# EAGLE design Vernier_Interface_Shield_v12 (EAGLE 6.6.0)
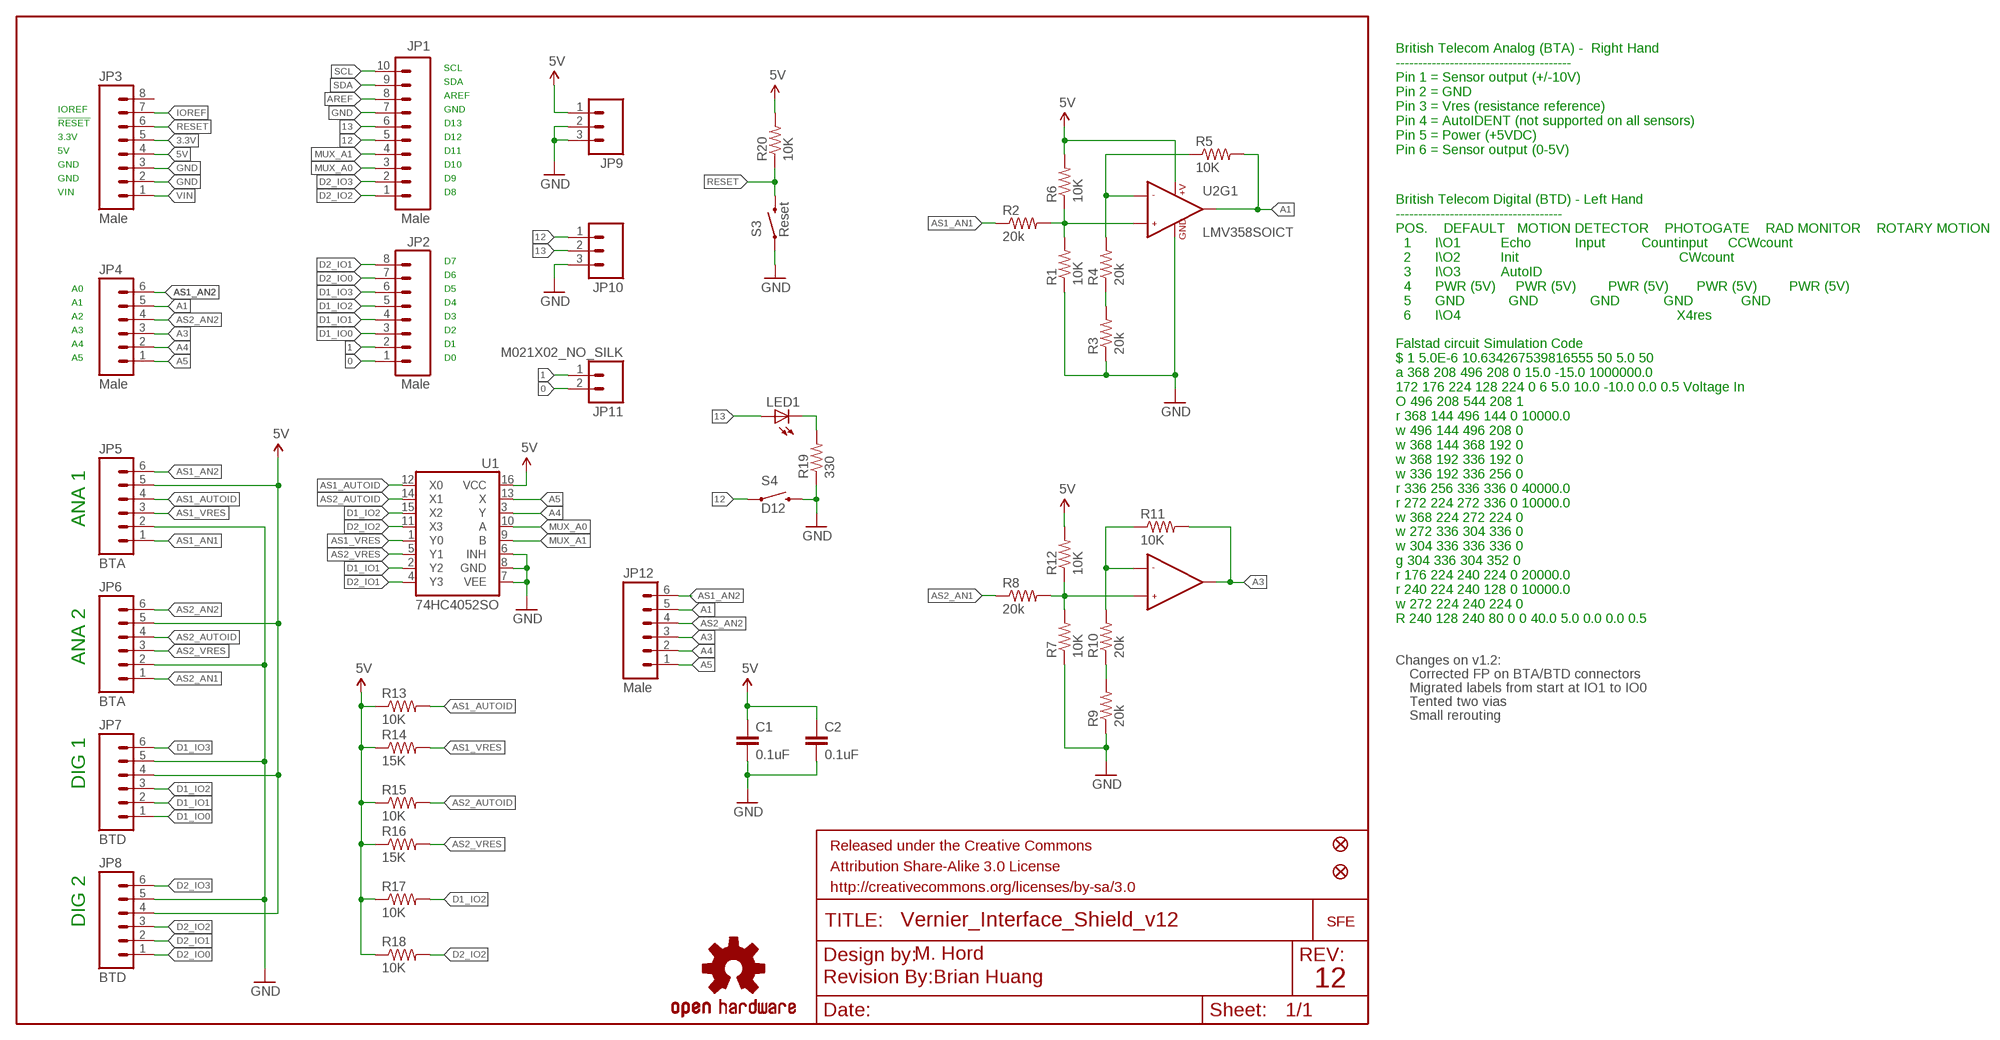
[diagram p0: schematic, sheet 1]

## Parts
C1  0.1uF  0.1UF-25V(+80/-20%)(0603)  [0603-CAP]
C2  0.1uF  0.1UF-25V(+80/-20%)(0603)  [0603-CAP]
FID1  FIDUCIAL1X2  [FIDUCIAL-1X2]
FID2  FIDUCIAL1X2  [FIDUCIAL-1X2]
FRAME1  FRAME-LETTER  [CREATIVE_COMMONS]
JP1  Male  M10SMD_MALE  [1X10_SMD_MALE]
JP2  Male  M08SMD-MALE  [1X08_SMD_MALE]
JP3  Male  M08SMD-MALE  [1X08_SMD_MALE]
JP4  Male  M06SMD_MALE  [1X06_SMD_MALE]
JP5  BTA  M06VERNIER-ANALOG  [BTA]
JP6  BTA  M06VERNIER-ANALOG  [BTA]
JP7  BTD  M06VERNIER-DIGITAL  [BTD]
JP8  BTD  M06VERNIER-DIGITAL  [BTD]
JP9  M031X03_NO_SILK  [1X03_NO_SILK]
JP10  M031X03_NO_SILK  [1X03_NO_SILK]
JP11  M021X02_NO_SILK  [1X02_NO_SILK]
JP12  Male  M06SIP  [1X06]
LED1  LED5MM  [LED5MM]
LOGO2  OSHW-LOGOS  [OSHW-LOGO-S]
LOGO_1  LOGO-SFESK  [SFE-LOGO-FLAME]
R1  10K  10KOHM1/10W1%(0603)0603  [0603-RES]
R2  20k  20KOHM1/10W1%(0603)  [0603-RES]
R3  20k  20KOHM1/10W1%(0603)  [0603-RES]
R4  20k  20KOHM1/10W1%(0603)  [0603-RES]
R5  10K  10KOHM1/10W1%(0603)0603  [0603-RES]
R6  10K  10KOHM1/10W1%(0603)0603  [0603-RES]
R7  10K  10KOHM1/10W1%(0603)0603  [0603-RES]
R8  20k  20KOHM1/10W1%(0603)  [0603-RES]
R9  20k  20KOHM1/10W1%(0603)  [0603-RES]
R10  20k  20KOHM1/10W1%(0603)  [0603-RES]
R11  10K  10KOHM1/10W1%(0603)0603  [0603-RES]
R12  10K  10KOHM1/10W1%(0603)0603  [0603-RES]
R13  10K  10KOHM1/10W1%(0603)0603  [0603-RES]
R14  15K  15KOHM1/10W1%(0603)0603  [0603-RES]
R15  10K  10KOHM1/10W1%(0603)0603  [0603-RES]
R16  15K  15KOHM1/10W1%(0603)0603  [0603-RES]
R17  10K  10KOHM1/10W1%(0603)0603  [0603-RES]
R18  10K  10KOHM1/10W1%(0603)0603  [0603-RES]
R19  330  330OHM1/10W1%(0603)  [0603-RES]
R20  10K  10KOHM1/10W1%(0603)0603  [0603-RES]
S3  Reset  SWITCH-MOMENTARY-2PTH  [TACTILE-PTH]
S4  D12  SWITCH-MOMENTARY-2PTH  [TACTILE-PTH]
U1  74HC4052SO  [SO16]
U2  LMV358SOICT  [SO08-TIGHT]
U$1  REVISION  [REVISION]

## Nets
0: JP2.1 JP11.2
1: JP2.2 JP11.1
3.3V: JP3.5
5V: C1.1 C2.1 JP3.4 JP5.5 JP6.5 JP7.4 JP8.4 JP9.1 R6.2 R12.2 R13.1 R14.1 R15.1 R16.1 R17.1 R18.1 R20.2 U1.16(VCC) U2.8(+V)
12: JP1.5 JP10.1 S4.1
13: JP1.6 JP10.2 LED1.A
A1: JP4.5 JP12.5 R5.2 U2.1(OUT1)
A3: JP4.3 JP12.3 R11.2 U2.7(OUT2)
A4: JP4.2 JP12.2 U1.3(Y)
A5: JP4.1 JP12.1 U1.13(X)
AREF: JP1.8
AS1_AN1: JP5.1 R2.1
AS1_AN2: JP4.6 JP5.6 JP12.6
AS1_AUTOID: JP5.4 R13.2 U1.12(X0)
AS1_VRES: JP5.3 R14.2 U1.1(Y0)
AS2_AN1: JP6.1 R8.1
AS2_AN2: JP4.4 JP6.6 JP12.4
AS2_AUTOID: JP6.4 R15.2 U1.14(X1)
AS2_VRES: JP6.3 R16.2 U1.5(Y1)
D1_IO0: JP2.3 JP7.1
D1_IO1: JP2.4 JP7.2 U1.2(Y2)
D1_IO2: JP2.5 JP7.3 R17.2 U1.15(X2)
D1_IO3: JP2.6 JP7.6
D2_IO0: JP2.7 JP8.1
D2_IO1: JP2.8 JP8.2 U1.4(Y3)
D2_IO2: JP1.1 JP8.3 R18.2 U1.11(X3)
D2_IO3: JP1.2 JP8.6
GND: C1.2 C2.2 JP1.7 JP3.2 JP3.3 JP5.2 JP6.2 JP7.5 JP8.5 JP9.2 JP9.3 JP10.3 R1.1 R3.1 R7.1 R9.1 R19.1 S3.1 S4.3 U1.6(INH) U1.7(VEE) U1.8(GND) U2.4(GND)
IOREF: JP3.7
MUX_A0: JP1.3 U1.10(A)
MUX_A1: JP1.4 U1.9(B)
N$1: R1.2 R2.2 R6.1 U2.3(+IN1)
N$2: R3.2 R4.1
N$3: R4.2 R5.1 U2.2(-IN1)
N$5: R9.2 R10.1
N$6: R7.2 R8.2 R12.1 U2.5(+IN2)
N$8: R10.2 R11.1 U2.6(-IN2)
N$9: LED1.K(C) R19.2
RESET: JP3.6 R20.1 S3.3
SCL: JP1.10
SDA: JP1.9
VIN: JP3.1
Unconnected: JP3.8

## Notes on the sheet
- SCL
- SDA
- AREF
- IOREF | GND
- !RESET | D13
- 3.3V | D12
- 5V | D11
- British Telecom Analog (BTA) -  Right Hand
  ---------------------------------------
  Pin 1 = Sensor output (+/-10V)
  Pin 2 = GND
  Pin 3 = Vres (resistance reference)
  Pin 4 = AutoIDENT (not supported on all sensors)
  Pin 5 = Power (+5VDC)
  Pin 6 = Sensor output (0-5V)
- GND | D10
- GND | D9
- VIN | D8
- D7
- D6
- A0 | D5
- A1 | D4
- A2 | D3
- British Telecom Digital (BTD) - Left Hand
  -------------------------------------
  POS.    DEFAULT   MOTION DETECTOR    PHOTOGATE    RAD MONITOR    ROTARY MOTION
    1      I\\O1          Echo           Input         Countinput     CCWcount 
    2      I\\O2          Init                                        CWcount 
    3      I\\O3          AutoID            
    4      PWR (5V)     PWR (5V)        PWR (5V)       PWR (5V)        PWR (5V)
    5      GND           GND             GND           GND            GND
    6      I\\O4                                                      X4res
- A3 | D2
- A4 | D1
- A5 | D0
- ANA 1
- Falstad circuit Simulation Code
  $ 1 5.0E-6 10.634267539816555 50 5.0 50
  a 368 208 496 208 0 15.0 -15.0 1000000.0
  172 176 224 128 224 0 6 5.0 10.0 -10.0 0.0 0.5 Voltage In
  O 496 208 544 208 1
  r 368 144 496 144 0 10000.0
  w 496 144 496 208 0
  w 368 144 368 192 0
  w 368 192 336 192 0
  w 336 192 336 256 0
  r 336 256 336 336 0 40000.0
  r 272 224 272 336 0 10000.0
  w 368 224 272 224 0
  w 272 336 304 336 0
  w 304 336 336 336 0
  g 304 336 304 352 0
  r 176 224 240 224 0 20000.0
  r 240 224 240 128 0 10000.0
  w 272 224 240 224 0
  R 240 128 240 80 0 0 40.0 5.0 0.0 0.0 0.5
- ANA 2 | Changes on v1.2:
- Corrected FP on BTA/BTD connectors
- Migrated labels from start at IO1 to IO0
- Tented two vias
- Small rerouting
- DIG 1
- DIG 2
- M. Hord
- Brian Huang | 12

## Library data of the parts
C1 C2 = SparkFun-Capacitors:0.1UF-25V(+80/-20%)(0603): CAP-00810; PROD_ID: CAP-00810
FID1 FID2 = SparkFun-Aesthetics:FIDUCIAL: Fiducial Alignment Points
FRAME1 = SparkFun-Aesthetics:FRAME-LETTER: Schematic Frame
JP1 = SparkFun-Connectors:M10: Header 10 Standard 10-pin 0.1" header. Use with straight break away headers (SKU : PRT-00116), right angle break away headers (PRT-00553), swiss pins (PRT-00743), machine pins (PRT-00117), and female headers (PRT-00115).; PROD_ID: CONN-11291
JP2 JP3 = SparkFun-Connectors:M08: Header 8 Standard 8-pin 0.1" header. Use with straight break away headers (SKU : PRT-00116), right angle break away headers (PRT-00553), swiss pins (PRT-00743), machine pins (PRT-00117), and female headers (PRT-00115).; PROD_ID: CONN-11292
JP4 = SparkFun-Connectors:M06: Header 6 Standard 6-pin 0.1" header. Use with straight break away headers (SKU : PRT-00116), right angle break away headers (PRT-00553), swiss pins (PRT-00743), machine pins (PRT-00117), and female headers (PRT-00115). Molex polarized connector foot print use with SKU : PRT-08094 with associated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; PROD_ID: CONN-11293
JP5-JP8 JP12 = SparkFun-Connectors:M06: Header 6 Standard 6-pin 0.1" header. Use with straight break away headers (SKU : PRT-00116), right angle break away headers (PRT-00553), swiss pins (PRT-00743), machine pins (PRT-00117), and female headers (PRT-00115). Molex polarized connector foot print use with SKU : PRT-08094 with associated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
JP9 JP10 = SparkFun-Connectors:M03: Header 3 Standard 3-pin 0.1" header. Use with straight break away headers (SKU : PRT-00116), right angle break away headers (PRT-00553), swiss pins (PRT-00743), machine pins (PRT-00117), and female headers (PRT-00115). Molex polarized connector foot print use with SKU : PRT-08232 with associated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
JP11 = SparkFun-Connectors:M02: Standard 2-pin 0.1" header. Use with
LED1 = SparkFun-LED:LED: LEDs
LOGO2 = SparkFun-Aesthetics:OSHW-LOGO: Open Source Hardware Logo This logo indicates the piece of hardware it is found on incorporates a OSHW license and/or adheres to the definition of open source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
LOGO_1 = SparkFun-Aesthetics:LOGO-SFE: Spark Fun Electronics PCB Logo
R1 R5-R7 R11-R13 R15 R17 R18 R20 = SparkFun-Resistors:10KOHM1/10W1%(0603): RES-00824; PROD_ID: RES-00824
R2-R4 R8-R10 = SparkFun-Resistors:20KOHM1/10W1%(0603): RES-09383; PROD_ID: RES-09383
R14 R16 = SparkFun-Resistors:15KOHM1/10W1%(0603): RES-07854; PROD_ID: RES-07854
R19 = SparkFun-Resistors:330OHM1/10W1%(0603): RES-00818; PROD_ID: RES-00818
S3 S4 = SparkFun-Electromechanical:SWITCH-MOMENTARY-2: Various NO switches- pushbuttons, reed, etc
U1 = SparkFun-AnalogIC:74HC4052: Dual 4:1 analog mux; PROD_ID: IC-09813; VALUE: 74HC4052
U2 = SparkFun-AnalogIC:LMV358: Jellybean rail-to-rail output op-amp; PROD_ID: IC-09657
U$1 = SparkFun-Aesthetics:REVISION

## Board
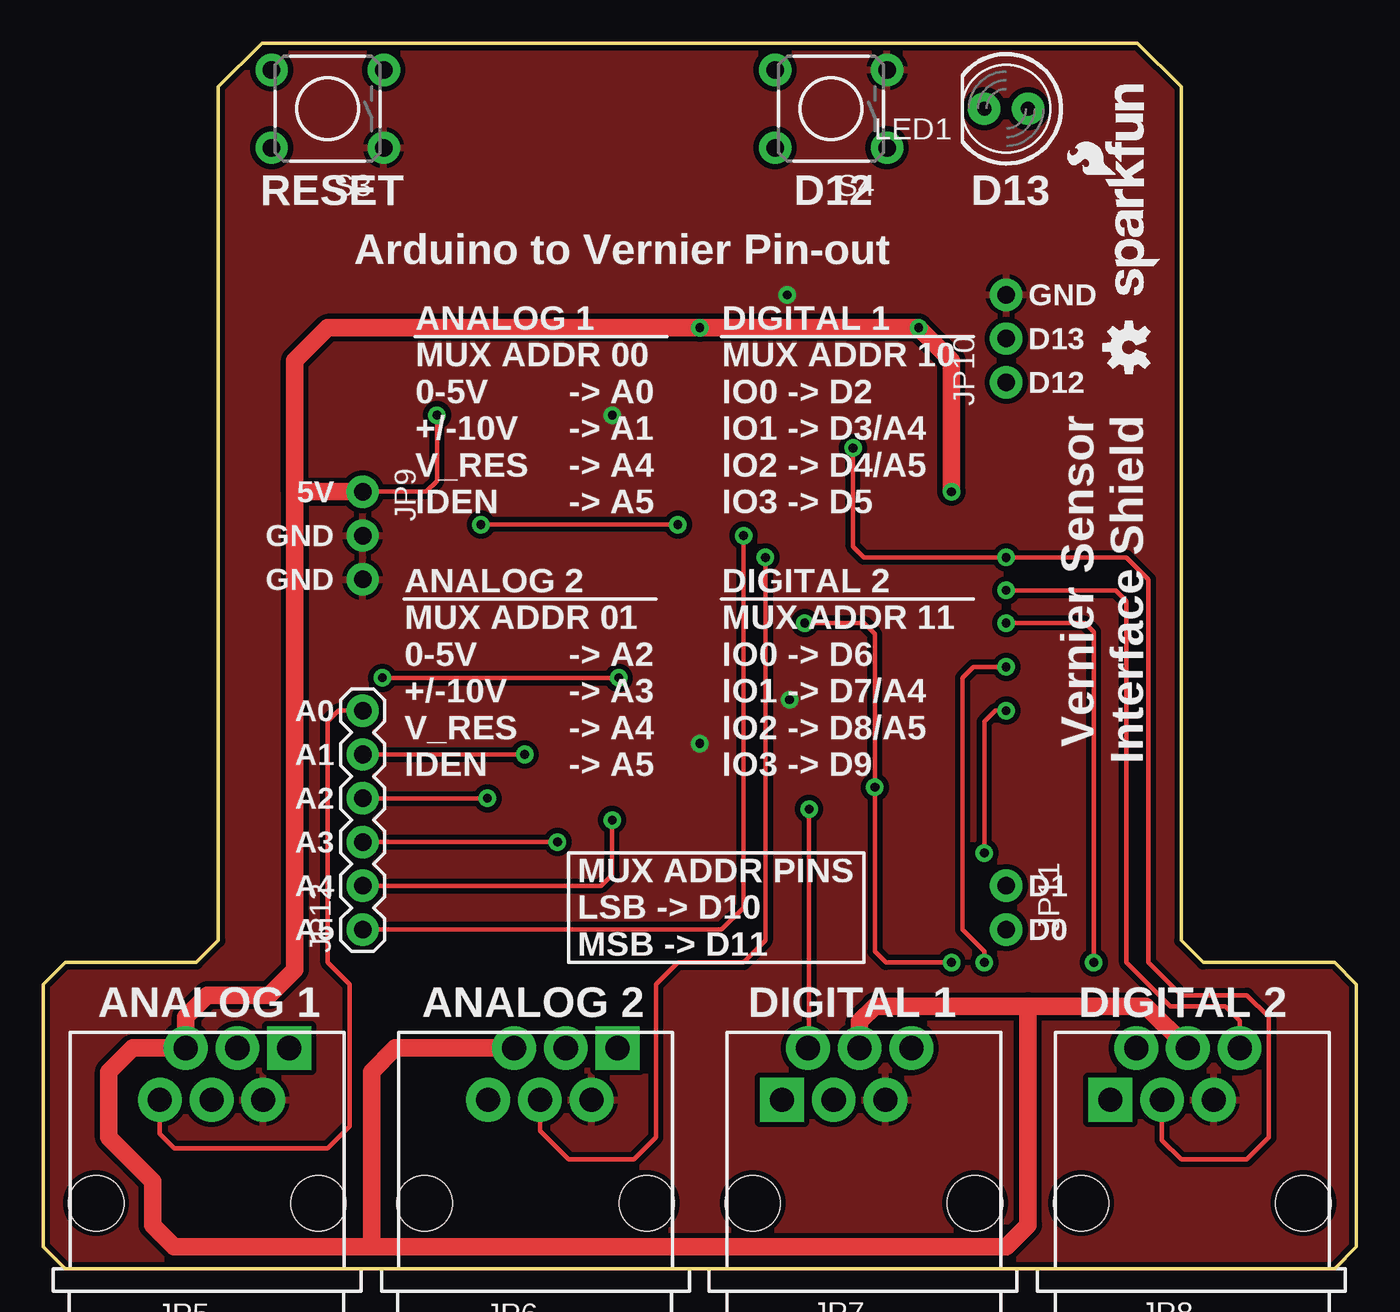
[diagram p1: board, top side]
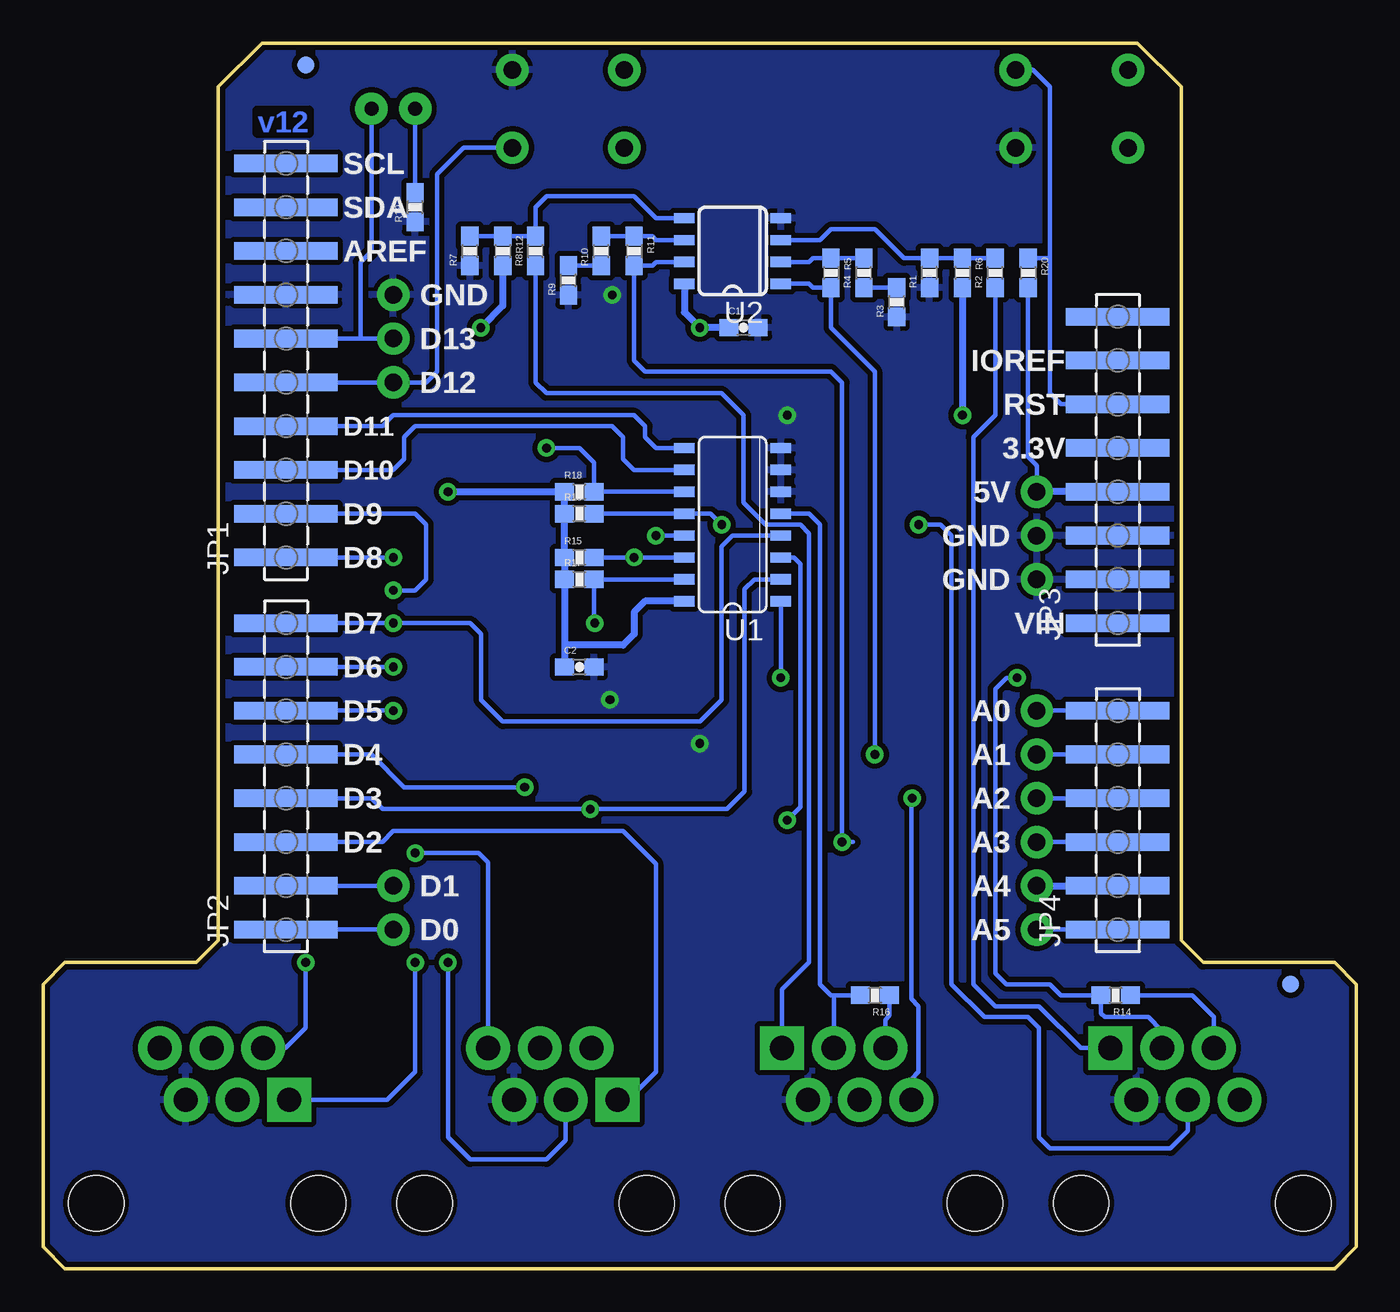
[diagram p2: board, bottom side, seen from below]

Size 76.2 x 71.12 mm. Coordinates in mm from the lower left corner, seen from the top.
Outline: 1.27,0 74.93,0 76.2,1.27 76.2,16.51 74.93,17.78 67.31,17.78 66.04,19.05 66.04,68.58 63.5,71.12 12.7,71.12 10.16,68.58 10.16,19.05 8.89,17.78 1.27,17.78 0,16.51 0,1.27 1.27,0
Copper layers (1*16): Top 0.035mm / dielectric 1.5mm / Bottom 0.035mm
Design rules "SparkFun-2-layer": minimum track width 7mil, minimum drill 15mil, track to track 8mil, track to pad 8mil, pad to pad 8mil, via to via 8mil, smd to smd 8mil, copper to edge 8mil, drill to drill 8mil, minimum pad ring 12mil, minimum via ring 10mil, stop-mask expansion 4mil, vias tented up to drill 20mil, thermal gap 10mil

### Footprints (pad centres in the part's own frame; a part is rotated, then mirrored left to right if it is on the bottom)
0603-CAP = smd 1.1 x 1: 1 -0.85,0; 2 0.85,0
FIDUCIAL-1X2 = smd 1 x 1: 1 0,0
1X10_SMD_MALE = smd 1.02 x 6: 1 0,0; 2 2.54,0; 3 5.08,0; 4 7.62,0; 5 10.16,0; 6 12.7,0; 7 15.24,0; 8 17.78,0; 9 20.32,0; 10 22.86,0
1X08_SMD_MALE = smd 1.02 x 6: 1 0,0; 2 2.54,0; 3 5.08,0; 4 7.62,0; 5 10.16,0; 6 12.7,0; 7 15.24,0; 8 17.78,0
1X06_SMD_MALE = smd 1.02 x 6: 1 0,0; 2 2.54,0; 3 5.08,0; 4 7.62,0; 5 10.16,0; 6 12.7,0
BTA = drill 1.4 pad 2.54 square: 1 4.75,9 | drill 1.4 pad 2.54: 2 3.25,6; 3 1.75,9; 4 0.25,6; 5 -1.25,9; 6 -2.75,6 | hole 3.2: 6.45,0; -6.45,0
BTD = drill 1.4 pad 2.54 square: 1 -4.75,6 | drill 1.4 pad 2.54: 2 -3.25,9; 3 -1.75,6; 4 -0.25,9; 5 1.25,6; 6 2.75,9 | hole 3.2: 6.45,0; -6.45,0
1X03_NO_SILK = drill 1.016 pad 1.88: 1 0,0; 2 2.54,0; 3 5.08,0
1X02_NO_SILK = drill 1.016 pad 1.88: 1 0,0; 2 2.54,0
1X06 = drill 1.016 pad 1.88: 1 0,0; 2 2.54,0; 3 5.08,0; 4 7.62,0; 5 10.16,0; 6 12.7,0
LED5MM = drill 0.813 pad 1.88: A -1.27,0; K 1.27,0
0603-RES = smd 1.1 x 1: 1 -0.85,0; 2 0.85,0
TACTILE-PTH = drill 1.016 pad 1.88: 1 -3.251,2.261; 2 3.251,2.261; 3 -3.251,-2.261; 4 3.251,-2.261
SO16 = smd 0.6 x 1.2: 1 -4.445,-2.8; 2 -3.175,-2.8; 3 -1.905,-2.8; 4 -0.635,-2.8; 5 0.635,-2.8; 6 1.905,-2.8; 7 3.175,-2.8; 8 4.445,-2.8; 9 4.445,2.8; 10 3.175,2.8; 11 1.905,2.8; 12 0.635,2.8; 13 -0.635,2.8; 14 -1.905,2.8; 15 -3.175,2.8; 16 -4.445,2.8
SO08-TIGHT = smd 0.6 x 1.2: 1 -1.905,-2.8; 2 -0.635,-2.8; 3 0.635,-2.8; 4 1.905,-2.8; 5 1.905,2.8; 6 0.635,2.8; 7 -0.635,2.8; 8 -1.905,2.8

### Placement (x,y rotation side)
C1  35.56,54.61 0 bottom
C2  45.09,34.92 0 bottom
FID1  3.81,16.51 0 bottom
FID2  60.96,69.85 0 bottom
FRAME1  not placed on the board
JP1  62.1,41.27 90 bottom
JP2  62.1,19.68 90 bottom
JP3  13.84,37.47 90 bottom
JP4  13.84,19.68 90 bottom
JP5  9.53,3.81 0 top
JP6  28.57,3.81 0 top
JP7  47.62,3.81 0 top
JP8  66.67,3.81 0 top
JP9  18.54,45.09 270 top
JP10  55.88,51.44 90 top
JP11  55.88,22.23 270 top
JP12  18.54,19.68 90 top
LED1  55.88,67.31 180 top
LOGO2  62.99,53.47 90 top
LOGO_1  62.23,63.5 90 top
LOGO_3  LOGO-SFENW2  [SFE-NEW-WEB]  64.77,56.52 90 top
R1  24.77,57.78 90 bottom
R2  20.95,57.78 90 bottom
R3  26.67,56.08 90 bottom
R4  28.57,57.78 90 bottom
R5  30.48,57.78 270 bottom
R6  22.86,57.78 270 bottom
R7  51.44,59.05 90 bottom
R8  47.62,59.05 90 bottom
R9  45.72,57.35 90 bottom
R10  43.81,59.05 90 bottom
R11  41.91,59.05 270 bottom
R12  49.53,59.05 270 bottom
R13  45.09,43.81 0 bottom
R14  13.97,15.88 180 bottom
R15  45.09,41.27 0 bottom
R16  27.94,15.88 180 bottom
R17  45.09,40.01 0 bottom
R18  45.09,45.09 0 bottom
R19  54.61,61.59 90 bottom
R20  19.05,57.78 270 bottom
S3  16.51,67.31 180 top
S4  45.72,67.31 180 top
U1  36.2,43.18 90 bottom
U2  36.2,59.05 90 bottom
U$1  not placed on the board

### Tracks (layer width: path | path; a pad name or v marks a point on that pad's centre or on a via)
0
  Bottom 0.254: JP2.1 JP11.2
1
  Bottom 0.254: JP2.2 JP11.1
5V  (via drill 0.51)
  Top 0.254: JP9.1 22.23,45.09 22.86,45.72 v22.86,49.53
  Top 1.016: 14.61,45.09 JP9.1 | 57.15,15.24 48.26,15.24 47.38,14.36 JP7.4 | 57.15,15.24 63.99,15.24 JP8.4 | JP6.5 20.43,12.81 19.05,11.43 19.05,1.27 | 19.05,1.27 7.62,1.27 6.35,2.54 6.35,5.08 3.81,7.62 3.81,11.43 5.19,12.81 JP5.5 8.28,14.62 9.53,15.88 R14.1 14.61,17.36 14.61,45.09 | 19.05,1.27 55.88,1.27 57.15,2.54 57.15,15.24 | 14.61,45.09 14.61,52.7 16.51,54.61 v38.1,54.61 v50.8,54.61 52.7,52.7 v52.7,45.09
  Bottom 0.254: R14.1 9.53,15.88 8.28,14.62 JP5.5 | JP6.5 27.32,14.46 27.09,14.69 R16.1 | R20.2 19.05,47.12 18.54,46.61 JP9.1
  Bottom 0.406: 45.94,36.2 R17.1 R15.1 R13.1 R18.1 v52.7,45.09 | 45.94,36.2 C2.1 | U1.16 41.27,38.73 41.91,38.1 41.91,36.83 42.55,36.2 45.94,36.2 | R6.2 v22.86,49.53 | C1.1 v38.1,54.61 38.99,55.51 U2.8 | JP3.4 JP9.1 | R12.2 49.53,55.88 v50.8,54.61
12
  Bottom 0.254: JP1.5 JP10.1 53.98,51.44 53.34,52.07 53.34,63.5 51.79,65.05 S4.1
13
  Bottom 0.254: JP1.6 57.78,53.98 | 57.78,53.98 JP10.2 | LED1.A 57.15,59.05 57.78,58.42 57.78,53.98
A1  (via drill 0.51)
  Top 0.254: JP12.5 v27.94,29.84
  Bottom 0.254: v27.94,29.84 27.94,52.07 30.48,54.61 R5.2 31.54,56.94 31.75,57.15 U2.1 | JP4.5 JP12.5
A3  (via drill 0.51)
  Top 0.254: JP12.3 v29.84,24.77
  Bottom 0.254: U2.7 40.64,58.42 40.85,58.2 R11.2 41.91,52.7 41.27,52.07 30.48,52.07 29.84,51.44 v29.84,24.77 29.21,24.77 | JP4.3 JP12.3
A4  (via drill 0.51)
  Top 0.254: JP12.2 32.38,22.23 33.02,22.86 v33.02,26.04
  Bottom 0.254: U1.3 32.64,41.27 32.26,40.89 32.26,26.8 v33.02,26.04
  Bottom 0.406: JP12.2 JP4.2
A5  (via drill 0.51)
  Top 0.254: v40.64,42.55 40.64,20.95 39.37,19.68 JP12.1
  Bottom 0.254: U1.13 v40.64,42.55 | JP12.1 JP4.1
AS1_AN1
  Bottom 0.254: R2.1 20.95,49.53 22.23,48.26 22.23,16.51 20.95,15.24 18.41,15.24 15.98,12.81 JP5.1
AS1_AN2
  Top 0.254: JP5.6 6.78,7.83 7.62,6.99 16.51,6.99 17.78,8.26 17.78,16.51 16.51,17.78 16.51,31.75 17.14,32.38 JP12.6
  Bottom 0.254: JP12.6 JP4.6
AS1_AUTOID  (via drill 0.51)
  Top 0.254: v36.83,43.18 v25.4,43.18
  Bottom 0.254: R13.2 U1.12 37.47,43.81 v36.83,43.18 | JP5.4 9.78,8.01 10.79,6.99 17.78,6.99 18.41,7.62 18.41,13.97 19.05,14.61 21.59,14.61 23.5,16.51 23.5,42.55 24.13,43.18 v25.4,43.18
AS1_VRES  (via drill 0.51)
  Top 0.254: v19.68,34.29 v33.4,34.29
  Bottom 0.254: JP5.3 11.28,13.81 12.06,14.61 14.61,14.61 14.82,14.82 R14.2 17.14,15.88 17.78,16.51 20.32,16.51 20.95,17.14 20.95,33.66 20.32,34.29 v19.68,34.29 | U1.1 v33.4,34.3 v33.4,34.29
AS2_AN1
  Bottom 0.254: R8.1 47.62,51.44 46.99,50.8 36.83,50.8 35.56,49.53 35.56,44.45 34.29,43.18 32.26,43.18 31.75,42.67 31.75,17.78 33.33,16.2 JP6.1
AS2_AN2  (via drill 0.51)
  Top 0.254: JP12.4 v25.78,27.3
  Bottom 0.254: JP4.4 JP12.4 | v25.78,27.3 25.82,27.26 25.82,15.66 25.4,15.24 25.4,11.43 25.82,11.01 JP6.6
AS2_AUTOID  (via drill 0.51)
  Top 0.254: v41.91,41.27 41.91,19.05 40.64,17.78 36.83,17.78 35.56,16.51 35.56,7.62 34.29,6.35 30.48,6.35 28.82,8.01 JP6.4
  Bottom 0.254: R15.2 v41.91,41.27 U1.14
AS2_VRES
  Bottom 0.254: U1.5 31.75,43.81 31.11,43.18 31.11,16.51 30.48,15.88 30.35,15.88 | R16.2 30.35,15.88 | JP6.3 30.32,15.85 30.35,15.88
D1_IO0
  Bottom 0.254: JP7.1 42.26,9.81 40.64,11.43 40.64,23.5 42.55,25.4 55.88,25.4 56.52,24.77 JP2.3
D1_IO1  (via drill 0.51)
  Top 0.254: v44.45,26.67 44.45,12.88 JP7.2
  Bottom 0.254: U1.2 34.92,40.01 35.5,39.43 35.5,27.69 36.52,26.67 v44.45,26.67 56.52,26.67 57.15,27.3 JP2.4
D1_IO2  (via drill 0.51)
  Top 0.254: v44.2,37.47 47.62,37.47 48.26,36.83 v48.26,27.94 48.26,18.41 48.9,17.78 v52.7,17.78
  Bottom 0.254: U1.15 R17.2 44.23,37.5 v44.2,37.47 | v48.26,27.94 55.24,27.94 57.15,29.84 JP2.5 | v52.7,17.78 52.7,7.62 51.44,6.35 46.99,6.35 45.88,7.46 JP7.3
D1_IO3  (via drill 0.51)
  Top 0.254: v54.61,24.13 54.61,31.75 55.24,32.38 v55.88,32.38
  Bottom 0.254: v55.88,32.38 JP2.6 | v54.61,24.13 50.93,24.13 50.38,23.58 JP7.6
D2_IO0  (via drill 0.51)
  Top 0.254: v54.61,17.78 54.61,18.41 53.34,19.68 53.34,34.29 53.98,34.92 v55.88,34.92
  Bottom 0.254: JP2.7 v55.88,34.92 | JP8.1 56.23,9.81 54.61,11.43 v54.61,17.78
D2_IO1  (via drill 0.51)
  Top 0.254: v60.96,17.78 60.96,36.96 60.45,37.47 v55.88,37.47
  Bottom 0.254: JP8.2 62.12,12.81 60.96,13.97 v60.96,17.78 | U1.4 36.2,42.55 36.83,41.91 36.83,33.02 38.1,31.75 49.53,31.75 50.8,33.02 50.8,36.83 51.44,37.47 v55.88,37.47 JP2.8
D2_IO2  (via drill 0.51)
  Top 0.254: JP8.3 64.92,7.46 66.04,6.35 69.85,6.35 71.12,7.62 71.12,14.61 69.85,15.88 66.04,15.88 64.14,17.78 64.14,40.01 62.87,41.27 v55.88,41.27 47.62,41.27 46.99,41.91 v46.99,47.62
  Bottom 0.254: U1.11 R18.2 44.23,46.77 45.09,47.62 v46.99,47.62 | JP1.1 v55.88,41.27
D2_IO3  (via drill 0.51)
  Top 0.254: v55.88,39.37 62.23,39.37 62.87,38.73 62.87,17.78 65.41,15.24 68.58,15.24 69.42,14.39 JP8.6
  Bottom 0.254: JP1.2 54.61,43.81 53.98,43.18 53.98,40.01 54.61,39.37 v55.88,39.37
GND  (via drill 0.51)
  other vias: 43.31,33.02 43.18,56.52 33.02,49.53 38.1,30.48
  pour Bottom (isolate 0.305): 10.16,68.58 12.7,71.12 63.5,71.12 66.04,68.58 66.04,19.05 67.31,17.78 74.93,17.78 76.2,16.51 76.2,1.27 74.93,0 1.27,0 0.13,1.14 0,1.14 0,16.51 1.27,17.78 8.89,17.78 10.16,19.05
  pour Top (isolate 0.305): 10.16,68.58 12.7,71.12 63.5,71.12 66.04,68.58 66.04,19.05 67.31,17.78 74.93,17.78 76.2,16.51 76.2,1.27 74.93,0 1.27,0 1.42,0.03 1.27,0.03 0,1.17 0,16.51 1.27,17.78 8.89,17.78 10.16,19.05
MUX_A0
  Bottom 0.254: U1.10 41.91,46.35 42.55,46.99 42.55,48.26 43.18,48.9 54.61,48.9 55.24,48.26 55.24,46.99 55.88,46.35 JP1.3
MUX_A1
  Bottom 0.254: U1.9 40.64,47.62 41.27,48.26 41.27,48.9 41.91,49.53 55.88,49.53 56.52,48.9 JP1.4
N$1
  Bottom 0.254: R2.2 R6.1 R1.2 26.25,58.63 27.94,60.33 30.48,60.33 31.11,59.69 U2.3
N$2
  Bottom 0.254: R4.1 R3.2
N$3
  Bottom 0.254: R4.2 R5.1 31.54,58.63 31.75,58.42 U2.2
N$5
  Bottom 0.254: R9.2 R10.1
N$6
  Bottom 0.254: U2.5 40.64,60.96 41.91,62.23 46.99,62.23 47.62,61.59 R8.2 R12.1 R7.2
N$8
  Bottom 0.254: U2.6 40.64,59.69 40.85,59.91 R11.1 R10.2
N$9
  Bottom 0.254: LED1.K R19.2
RESET
  Bottom 0.254: JP3.6 17.14,50.16 17.78,50.8 17.78,58.67 | 17.78,58.67 17.78,68.58 18.77,69.57 S3.3 | R20.1 17.82,58.63 17.78,58.67

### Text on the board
Bottom: v12
tPlace: RESET | D12 | D13 | Arduino to Vernier Pin-out | GND | D13 | D12 | Vernier Sensor / Interface Shield | 5V | ANALOG 1 / MUX ADDR 00 / 0-5V / +/-10V / V_RES / IDEN | -> A0 / -> A1 / -> A4 / -> A5 | DIGITAL 1 / MUX ADDR 10 / IO0 -> D2 / IO1 -> D3/A4 / IO2 -> D4/A5 / IO3 -> D5 | GND | GND | A0 | A1 | ANALOG 2 / MUX ADDR 01 / 0-5V / +/-10V / V_RES / IDEN | -> A2 / -> A3 / -> A4 / -> A5 | DIGITAL 2 / MUX ADDR 11 / IO0 -> D6 / IO1 -> D7/A4 / IO2 -> D8/A5 / IO3 -> D9 | A2 | A3 | A4 | D1 | A5 | D0 | MUX ADDR PINS / LSB -> D10 / MSB -> D11 | ANALOG 1 | ANALOG 2 | DIGITAL 1 | DIGITAL 2
bPlace: SCL | SDA | AREF | GND | D13 | IOREF | D12 | RST | D11 | 3.3V | D10 | 5V | D9 | GND | D8 | GND | VIN | D7 | D6 | A0 | D5 | A1 | D4 | A2 | D3 | A3 | D2 | A4 | D1 | A5 | D0
tDocu: M. Hord | Brian Huang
